(* Logix 5000 AddOnInstructionDefinition export AKD_Fault_Reset_Disable; software revision 19.01 *)

TYPE AKD_Status :   // All connections to the drive ethernet module are established and data is successfully transferring.
STRUCT
   Profile_In_Progress : BOOL;   // Profile Move In Progress
   Block_In_Execution : BOOL;   // Block In Execution
   On_Target_Position : BOOL;   // On Target Position (1=Current Position Equals Last Target Position)
   General_Fault : BOOL;   // General Fault
   Current_Direction : BOOL;   // Current Motor Direction (0=Reverse, 1=Forward)
   Home_Level : BOOL;   // Level of Home Input
   Reg_Level : BOOL;   // Level of Registration Input
   Enable : BOOL;   // State of Enable Output
   Fault_Input_Fault : BOOL;   // Fault Input Active
   Fwd_Limit : BOOL;   // Forward Input Active
   Rev_Limit : BOOL;   // Reverse Input Active
   Positive_Limit : BOOL;   // Positive Software Limit Exceeded
   Negative_Limit : BOOL;   // Negative Software Limit Exceeded
   FE_Fault : BOOL;   // Following Error Fault
   Block_Fault : BOOL;   // Block Execution Fault
   Load_Complete : BOOL;   // Command Message Successfully Loaded
END_STRUCT
END_TYPE

TYPE AKD_Control :   // Send Explicit Message
STRUCT
   Load_Data_Start_Profile : BOOL;   // Load Command Data / Start Profile Move
   Start_Block : BOOL;   // Execute Command block or block chain
   Incremental : BOOL;   // Incremental Position (0=Absolute, 1=Incremental)
   Direction : BOOL;   // Direction in Velocity Mode (0=Reverse, 1=Forward)
   Smooth_Stop : BOOL;   // Smooth / Controlled Stop w/ Deceleration
   Hard_Stop : BOOL;   // Hard / Immediate Stop
   Reg_Arm : BOOL;   // Arm the Registration Input
   Enable : BOOL;   // Enable Output
END_STRUCT
END_TYPE

TYPE AKD_Axis :   // Axis Data:
STRUCT
   Control : AKD_Control;   // Control bits to send to the drive
   Status : AKD_Status;   // Status bits received from the drive
   Input : AB:ETHERNET_MODULE_SINT_64Bytes:I:0;   // Data from the drive
   Output : AB:ETHERNET_MODULE_SINT_64Bytes:O:0;   // Data to the drive
   ResponseMsgType : SINT;   // Response type contained in latest IO response from drive. Used to check for errors
   CommandTimeout : INT;   // Time to allow for command response from drive. Dependent on scan rate and communicaiton rate
   PositionFeedback : DINT;   // Actual Position Value
   VelocityFeedback : DINT;   // Actual Velocity Value
END_STRUCT
END_TYPE

ADD_ON_INSTRUCTION AKD_Set_Parameter   (* revision 2.0, ExecutePrescan, ExecuteEnableInFalse *)
// Set Drive Parameter
VAR_OUTPUT
   DN : BOOL; {access Read Only, visible}   // Command Successful
   ER : BOOL; {access Read Only, visible}   // Error
END_VAR
VAR_IN_OUT
   Axis : AKD_Axis; {required}
END_VAR
VAR_INPUT
   Parameter_Number : INT; {visible}   // See help (F1) for parameter list.
   Parameter_Value : DINT; {required}   // Parameter Value
END_VAR
VAR
   Command_Timeout : TIMER := (PRE := 10000);   // Timeout Timer
   Command_Message_Type : SINT;   // Command Message Type
   Command_Axis_Number : SINT;   // Command Axis Number
   Step : SINT;
   Command_Bytes : SINT[8];
   OS_LoadStart : BOOL;
   Temp_Bytes : SINT[2];   // Temporary Bytes to Split into Command Bytes
END_VAR

ROUTINE EnableInFalse   (* ladder *)
// EnableIn_False
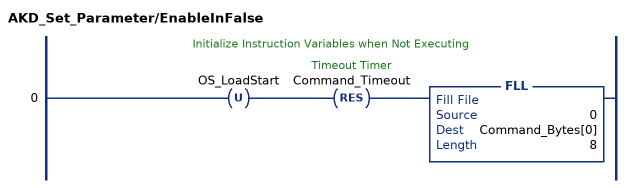
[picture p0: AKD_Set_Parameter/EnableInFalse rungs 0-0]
   // Initialize Instruction Variables when Not Executing
   0: OTU(OS_LoadStart)RES(Command_Timeout)FLL(0,Command_Bytes[0],8);
END_ROUTINE

ROUTINE Logic   (* ladder *)
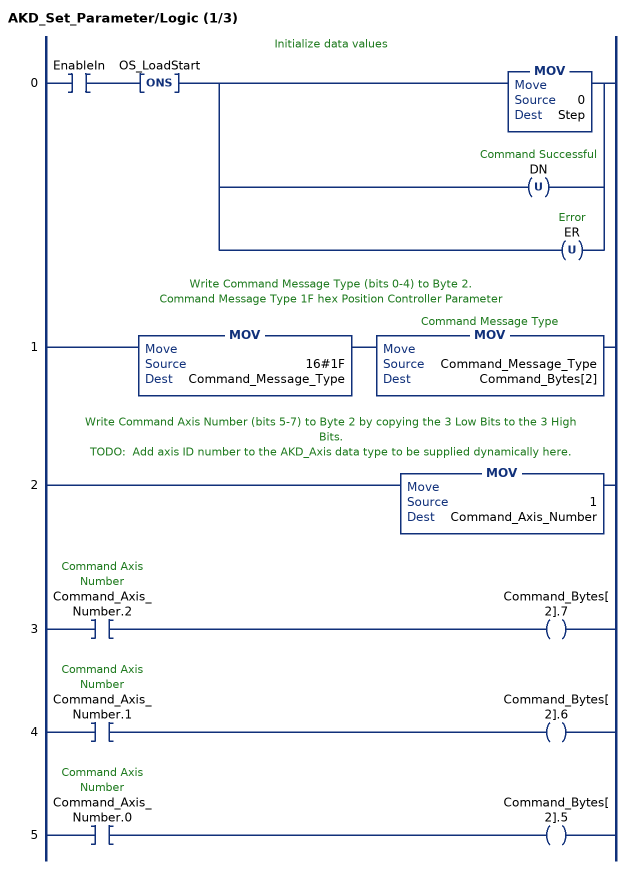
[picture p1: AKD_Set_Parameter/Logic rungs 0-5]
   // Initialize data values
   0: XIC(EnableIn)ONS(OS_LoadStart)[MOV(0,Step) ,OTU(DN) ,OTU(ER) ];
   // Write Command Message Type (bits 0-4) to Byte 2.
   // Command Message Type 1F hex Position Controller Parameter
   1: MOV(16#1F,Command_Message_Type)MOV(Command_Message_Type,Command_Bytes[2]);
   // Write Command Axis Number (bits 5-7) to Byte 2 by copying the 3 Low Bits to the 3 High Bits.
   // TODO:  Add axis ID number to the AKD_Axis data type to be supplied dynamically here.
   2: MOV(1,Command_Axis_Number);
   3: XIC(Command_Axis_Number.2)OTE(Command_Bytes[2].7);
   4: XIC(Command_Axis_Number.1)OTE(Command_Bytes[2].6);
   5: XIC(Command_Axis_Number.0)OTE(Command_Bytes[2].5);
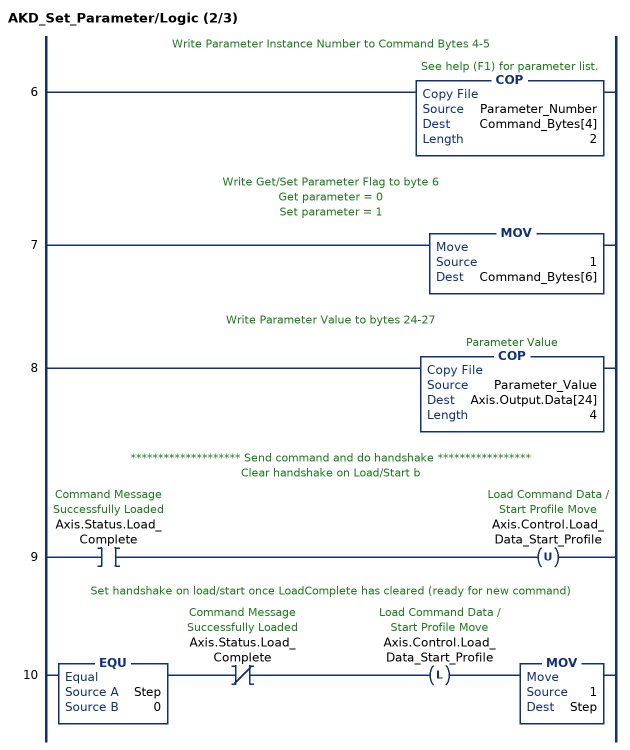
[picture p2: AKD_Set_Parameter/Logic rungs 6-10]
   // Write Parameter Instance Number to Command Bytes 4-5
   6: COP(Parameter_Number,Command_Bytes[4],2);
   // Write Get/Set Parameter Flag to byte 6
   // Get parameter = 0
   // Set parameter = 1
   7: MOV(1,Command_Bytes[6]);
   // Write Parameter Value to bytes 24-27
   8: COP(Parameter_Value,Axis.Output.Data[24],4);
   // ******************** Send command and do handshake *****************
   // Clear handshake on Load/Start b
   9: XIC(Axis.Status.Load_Complete)OTU(Axis.Control.Load_Data_Start_Profile);
   // Set handshake on load/start once LoadComplete has cleared (ready for new command)
   10: EQU(Step,0)XIO(Axis.Status.Load_Complete)OTL(Axis.Control.Load_Data_Start_Profile)MOV(1,Step);
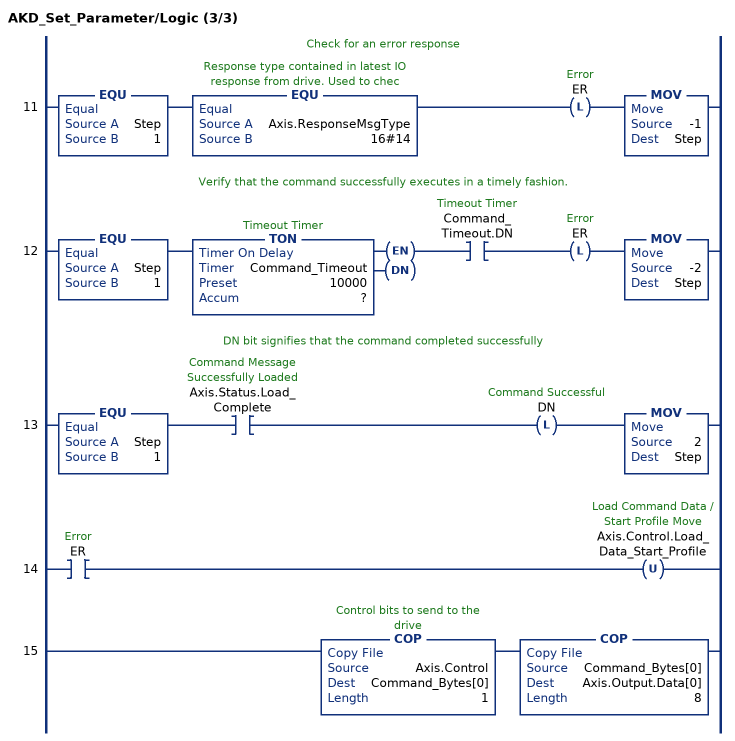
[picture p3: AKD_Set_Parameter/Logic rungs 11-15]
   // Check for an error response
   11: EQU(Step,1)EQU(Axis.ResponseMsgType,16#14)OTL(ER)MOV(-1,Step);
   // Verify that the command successfully executes in a timely fashion.
   12: EQU(Step,1)TON(Command_Timeout,?,?)XIC(Command_Timeout.DN)OTL(ER)MOV(-2,Step);
   // DN bit signifies that the command completed successfully
   13: EQU(Step,1)XIC(Axis.Status.Load_Complete)OTL(DN)MOV(2,Step);
   14: XIC(ER)OTU(Axis.Control.Load_Data_Start_Profile);
   15: COP(Axis.Control,Command_Bytes[0],1)COP(Command_Bytes[0],Axis.Output.Data[0],8);
END_ROUTINE

ROUTINE Prescan   (* ladder *)
// Prescan
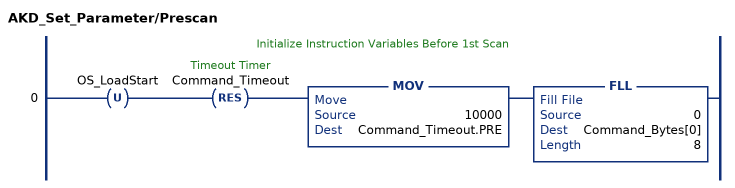
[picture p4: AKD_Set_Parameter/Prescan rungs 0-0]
   // Initialize Instruction Variables Before 1st Scan
   0: OTU(OS_LoadStart)RES(Command_Timeout)MOV(10000,Command_Timeout.PRE)FLL(0,Command_Bytes[0],8);
END_ROUTINE
END_ADD_ON_INSTRUCTION

ADD_ON_INSTRUCTION AKD_Fault_Reset_Disable   (* revision 2.0, ExecutePrescan, ExecuteEnableInFalse *)
// Drive Fault Reset & Disable
VAR_OUTPUT
   DN : BOOL; {access Read Only, visible}   // Command Successful
   ER : BOOL; {access Read Only, visible}   // Error
END_VAR
VAR_IN_OUT
   Axis : AKD_Axis; {required}
END_VAR
VAR
   Step : SINT;
   Set_Parameter : AKD_Set_Parameter := (Parameter_Number := 113);
END_VAR

ROUTINE EnableInFalse   (* ladder *)
// EnableIn_False
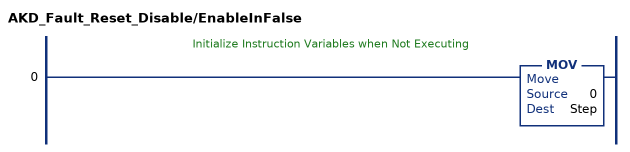
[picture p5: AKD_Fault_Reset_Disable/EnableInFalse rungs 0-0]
   // Initialize Instruction Variables when Not Executing
   0: MOV(0,Step);
END_ROUTINE

ROUTINE Logic   (* ladder *)
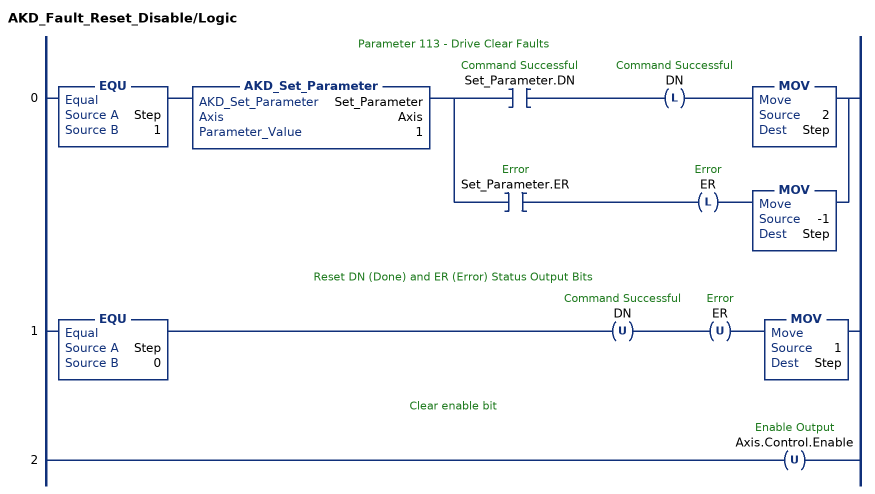
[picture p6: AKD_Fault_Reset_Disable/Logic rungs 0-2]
   // Parameter 113 - Drive Clear Faults
   0: EQU(Step,1)AKD_Set_Parameter(Set_Parameter,Axis,1)[XIC(Set_Parameter.DN) OTL(DN) MOV(2,Step) ,XIC(Set_Parameter.ER) OTL(ER) MOV(-1,Step) ];
   // Reset DN (Done) and ER (Error) Status Output Bits
   1: EQU(Step,0)OTU(DN)OTU(ER)MOV(1,Step);
   // Clear enable bit
   2: OTU(Axis.Control.Enable);
END_ROUTINE

ROUTINE Prescan   (* ladder *)
// Prescan
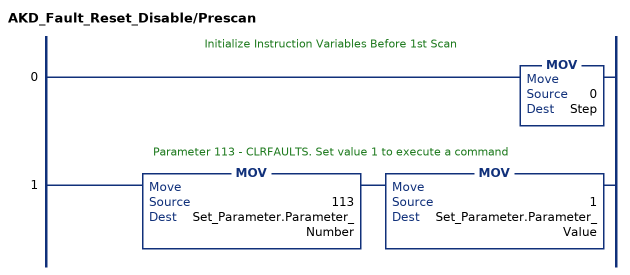
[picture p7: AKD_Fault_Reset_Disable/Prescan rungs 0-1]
   // Initialize Instruction Variables Before 1st Scan
   0: MOV(0,Step);
   // Parameter 113 - CLRFAULTS. Set value 1 to execute a command
   1: MOV(113,Set_Parameter.Parameter_Number)MOV(1,Set_Parameter.Parameter_Value);
END_ROUTINE
END_ADD_ON_INSTRUCTION
